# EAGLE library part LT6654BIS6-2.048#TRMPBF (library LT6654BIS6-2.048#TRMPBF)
LINEAR TECHNOLOGY - LT6654BIS6-2.048#TRMPBF - Voltage Reference, Series - Fixed, LT6654 Series, 2.048V reference, 0.1 %, +/- 10ppm/C, TSOT-23-6 Source: Datasheet
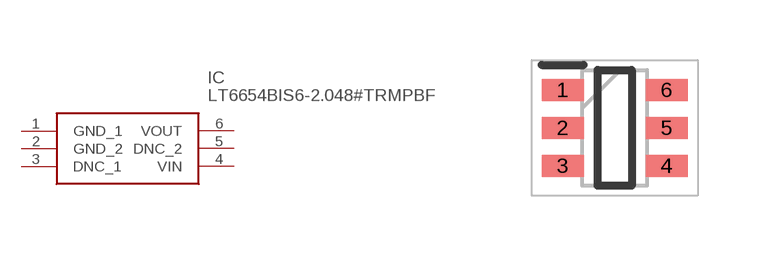
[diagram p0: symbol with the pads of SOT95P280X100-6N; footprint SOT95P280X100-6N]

Designator prefix IC

## LT6654BIS6-2.048#TRMPBF (Description: LINEAR TECHNOLOGY - LT6654BIS6-2.048#TRMPBF - Voltage Reference, Series - Fixed, LT6654 Series, 2.048V reference, 0.1 %, +/- 10ppm/C, TSOT-23-6; Height: 1mm; Manufacturer_Name: Analog Devices; Manufacturer_Part_Number: LT6654BIS6-2.048#TRMPBF)  [SOT95P280X100-6N]
1  GND_1
2  GND_2
3  DNC_1
4  VIN
5  DNC_2
6  VOUT

## Footprint SOT95P280X100-6N (pad centres in mm)
6-Lead Plastic TSOT-23
smd 1.05 x 0.55: 1 -1.3,0.95; 2 -1.3,0; 3 -1.3,-0.95; 4 1.3,-0.95; 5 1.3,0; 6 1.3,0.95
